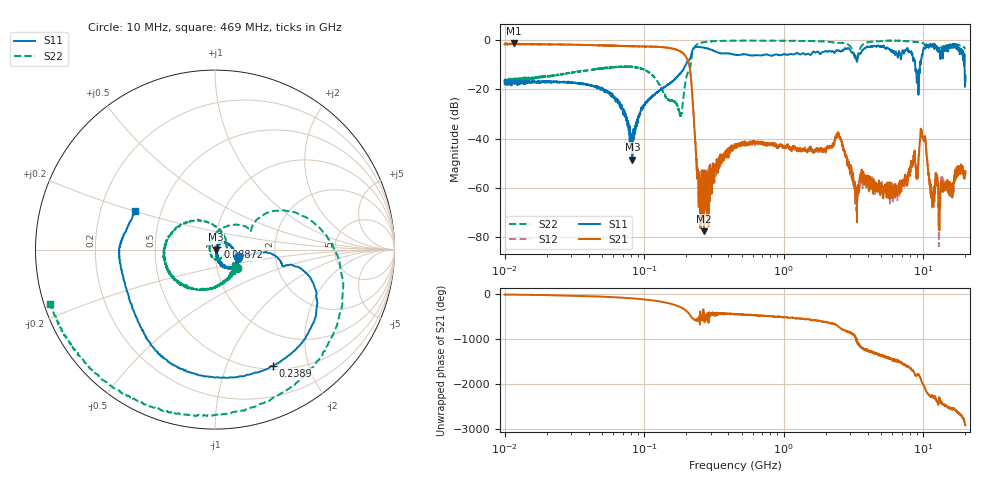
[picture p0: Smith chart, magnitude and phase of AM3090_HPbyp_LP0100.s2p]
# Hz S DB R 50
!freq MagS11 AngS11 MagS21 AngS21 MagS12 AngS12 MagS22 AngS22
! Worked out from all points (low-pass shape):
!   3201 points, 10 MHz to 20 GHz, reference 50 ohm
!   highest |S21| = -1.44 dB at 11.73 MHz (marker M1); lowest = -77.6 dB at 268.4 MHz (marker M2)
!   |S21| within 3 dB of the highest: start of sweep to 178.6 MHz
!   lowest |S11| = -48.4 dB at 82.23 MHz (marker M3), VSWR 1.01, Z = 50.4 - j0.00816 ohm
!   |S11| at or under -10 dB: start of sweep to 198.5 MHz; 8.73 GHz to 9.453 GHz (723.5 MHz wide, 7.96 % of centre); 19.73 GHz to end of sweep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
!   |S22| runs from -30.9 to -0.2 dB; largest |S21 - S12| = 0.03
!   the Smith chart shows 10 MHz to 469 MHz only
!   S11 on the Smith chart (normalised r, x): 10 MHz: 1.29, -0.12; 88.72 MHz: 1.03, +0.03; 238.9 MHz: 0.54, -1.48; 469 MHz: 0.35, +0.20
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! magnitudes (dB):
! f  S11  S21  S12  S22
! 10 MHz  -17.3  -1.8  -1.5  -16.1
! 11.73 MHz  -17.8  -1.4  -1.6  -16.4
! 35.55 MHz  -17.9  -2.0  -2.0  -12.7
! 61.1 MHz  -23.3  -2.4  -2.3  -11.0
! 82.23 MHz  -48.4  -2.5  -2.5  -11.0
! 88.72 MHz  -33.7  -2.6  -2.6  -11.3
! 126.1 MHz  -21.0  -2.8  -2.8  -17.4
! 180.9 MHz  -13.6  -4.6  -4.6  -30.9
! 205.2 MHz  -8.6  -8.2  -8.2  -13.3
! 218.3 MHz  -5.5  -18.0  -17.9  -7.1
! 238.9 MHz  -2.8  -51.5  -52.9  -1.9
! 268.4 MHz  -3.1  -77.6  -58.6  -0.9
! 447.2 MHz  -6.0  -43.4  -42.7  -0.3
! 469 MHz  -6.1  -43.1  -42.3  -0.3
! 1.59 GHz  -5.4  -44.4  -44.3  -0.4
! 2.444 GHz  -4.4  -37.5  -37.7  -1.3
! 3.297 GHz  -7.6  -63.8  -66.6  -8.2
! 5.639 GHz  -3.6  -60.5  -60.5  -0.3
! 9.025 GHz  -14.5  -56.1  -53.8  -0.9
! 9.831 GHz  -6.3  -38.8  -38.6  -1.2
! 11.58 GHz  -2.0  -62.5  -67.9  -2.1
! 20 GHz  -14.4  -54.0  -52.7  -3.7
